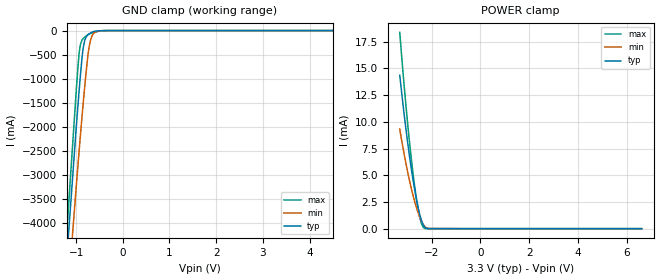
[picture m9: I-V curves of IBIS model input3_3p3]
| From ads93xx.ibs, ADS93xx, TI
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|   input3_3p3 Model
[Model]   input3_3p3
Model_type   Input
Vinl = 0.5
Vinh = 2.8
|   typ   min   max
C_comp   4.695pF   4.525pF   4.849pF
[Voltage Range]   3.3   3   3.5
[Temperature Range]   27   125   -40
[Power Clamp Reference]   3.3   3   3.5
[GND Clamp Reference]   0   0   0
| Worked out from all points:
|   GND clamp passes 1 mA (typ) near -0.41 V on its own axis
|   POWER clamp passes 1 mA (typ) near -2.44 V on its own axis
[GND Clamp]
|   Voltage   I(typ)   I(min)   I(max)
-3.3V     -26.03A    -23.71A    -28.8A
-1.34V    -6.704A    -7.567A    -6.354A
-1.191V   -4.628A    -5.679A    -4.088A
-1.162V   -4.218A    -5.3A      -3.641A
-1.003V   -2.092A    -3.317A    -1.337A
-933.9mV  -1.233A    -2.483A    -457mA
-864.6mV  -483.9mA   -1.689A    -184.6mA
-815.1mV  -206.5mA   -1.16A     -136.2mA
-726mV    -74.05mA   -371.9mA   -73.5mA
-646.8mV  -28.28mA   -88.08mA   -44.3mA
-369.6mV  -469.2uA   -442.7uA   -819.7uA
6.6V      0A         0A         0A
[POWER Clamp]
|   Voltage   I(typ)   I(min)   I(max)
-3.3V     14.37mA    9.321mA    18.38mA
-3.161V   11.51mA    7.497mA    14.5mA
-3.033V   9.066mA    5.943mA    11.18mA
-2.874V   6.359mA    4.232mA    7.542mA
-2.756V   4.565mA    3.106mA    5.153mA
-2.627V   2.871mA    2.047mA    2.95mA
-2.518V   1.676mA    1.294mA    1.471mA
-2.419V   828uA      738.7uA    533.2uA
-2.32V    276.8uA    330uA      88.67uA
-2.231V   58.62uA    107.5uA    6.401uA
-2.122V   3.563uA    12.69uA    513.2nA
6.6V      0A         0A         0A
